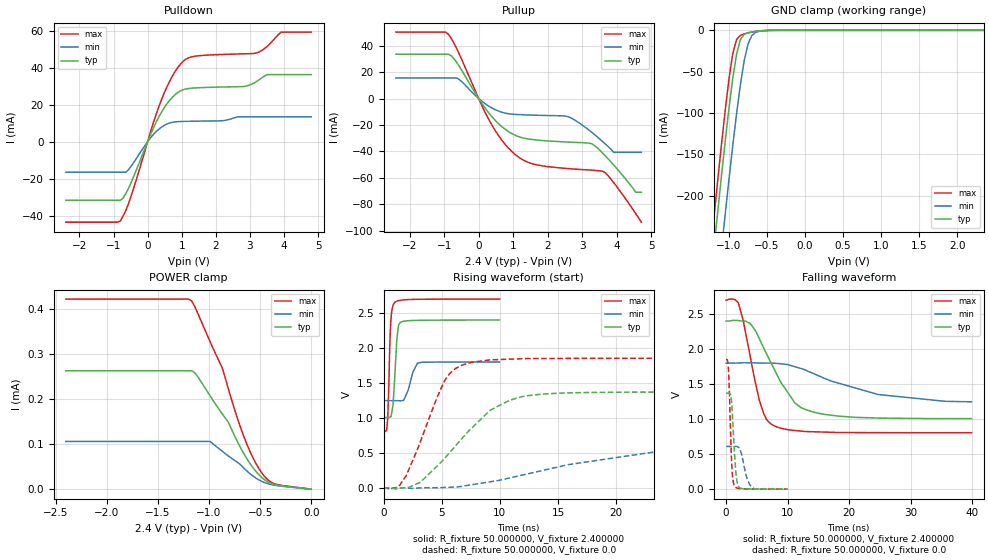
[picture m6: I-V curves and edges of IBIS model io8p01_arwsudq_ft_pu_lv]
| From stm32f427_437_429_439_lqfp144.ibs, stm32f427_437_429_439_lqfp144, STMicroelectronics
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|   Model io8p01_arwsudq_ft_pu_lv
[Model]  io8p01_arwsudq_ft_pu_lv
Model_type I/O
Polarity   Non-Inverting
Enable   Active-Low
Vinl =   0.720000V
Vinh =   1.680000V
Vmeas =  1.200000V
Cref =   50.000000pF
Rref =   100.000000M
Vref =   0.0V
C_comp   2.818400pF   2.774300pF   2.917100pF
[Temperature Range]   25.000000   0.125000k   -40.000000
[Pullup Reference]   2.400000V   1.800000V   2.700000V
[Pulldown Reference]   0.0V   0.0V   0.0V
[POWER Clamp Reference]   2.400000V   1.800000V   2.700000V
[GND Clamp Reference]   0.0V   0.0V   0.0V
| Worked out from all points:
|   slope of the pulldown table from 0 to 0.36 V, typ, clamps not added: 25 ohm
|   slope of the pullup table from 0 to 0.36 V, typ, clamps not added: 27.7 ohm
|   GND clamp passes 1 mA (typ) near -0.62 V on its own axis
|   rising waveform, R_fixture 50.000000, V_fixture 2.400000: 20-80 % time 290ps typ, 615ps min, 205ps max; typ from 1.01 V to 2.4 V
|   rising waveform, R_fixture 50.000000, V_fixture 0.0: 20-80 % time 4.71ns typ, 11.9ns min, 2.66ns max; typ from 0.001 V to 1.37 V
|   falling waveform, R_fixture 50.000000, V_fixture 2.400000: 20-80 % time 5.22ns typ, 11.3ns min, 2.74ns max; typ from 2.4 V to 1.01 V
|   falling waveform, R_fixture 50.000000, V_fixture 0.0: 20-80 % time 543ps typ, 1ns min, 410ps max; typ from 1.37 V to 0.001 V
[Pulldown]
|Voltage   I(typ)   I(min)   I(max)
-2.4V     -31.67mA   -16.51mA   -43.52mA
-800mV    -31.67mA   -16.51mA   -42.87mA
-480mV    -21.98mA   -13.17mA   -29.21mA
80mV      3.63mA     1.966mA    5.012mA
480mV     18.16mA    8.738mA    26.02mA
800mV     25.38mA    10.72mA    37.77mA
1.12V     28.53mA    11.02mA    44.6mA
2.8V      29.84mA    13.46mA    47.53mA
3.2V      32.6mA     13.46mA    48.03mA
3.52V     36.31mA    13.46mA    51.75mA
3.92V     36.31mA    13.46mA    59.29mA
4.8V      36.31mA    13.46mA    59.29mA
[Pullup]
|Voltage   I(typ)   I(min)   I(max)
-2.4V     33.5mA     15.56mA    50.23mA
-960mV    33.5mA     15.56mA    50.23mA
-560mV    24.27mA    14.3mA     33.51mA
320mV     -11.75mA   -6.207mA   -17.08mA
960mV     -26.47mA   -11.82mA   -40.02mA
1.52V     -30.88mA   -12.51mA   -49.05mA
2.56V     -32.88mA   -13.48mA   -52.9mA
3.28V     -34.19mA   -25.52mA   -54.17mA
3.6V      -41.32mA   -32.62mA   -54.98mA
3.92V     -50.33mA   -40.7mA    -63.65mA
4.56V     -70.9mA    -40.7mA    -87.11mA
4.72V     -70.9mA    -40.7mA    -93.5mA
[GND_clamp]
|Voltage   I(typ)   I(min)   I(max)
-2.4V     -1.425A    -1.509A    -1.395A
-1.25V    -311.8mA   -402mA     -274.5mA
-1.2V     -266mA     -356.2mA   -228.4mA
-1.15V    -220.9mA   -310.9mA   -183.1mA
-1.1V     -176.9mA   -266.3mA   -139mA
-1.05V    -134.3mA   -222.6mA   -97.01mA
-950mV    -57.81mA   -139.1mA   -27.86mA
-900mV    -28.73mA   -100.5mA   -11.04mA
-850mV    -11.29mA   -65.69mA   -6.054mA
-750mV    -2.852mA   -16.6mA    -3.179mA
-600mV    -750uA     -1.167mA   -738.5uA
2.35V     0A         0A         0A
[POWER_clamp]
|Voltage   I(typ)   I(min)   I(max)
-2.4V     263.2uA    106uA      422.4uA
-1.17V    263.2uA    106uA      418.5uA
-1.11V    250.1uA    106uA      391.1uA
-990mV    207.7uA    106uA      328.2uA
-870mV    167.2uA    84.17uA    269.6uA
-810mV    148.5uA    73.71uA    222.7uA
-660mV    79.21uA    47.09uA    117.6uA
-570mV    47.82uA    29.3uA     69.9uA
-510mV    31.66uA    20.4uA     45.18uA
-420mV    15.55uA    11.87uA    19.89uA
-360mV    10.34uA    8.845uA    12.09uA
0V        0A         0A         0A
[Ramp]
| variable   typ   min   max
dV/dt_r  0.82207/4.70989n   0.36536/11.91797n   1.11094/2.65517n
dV/dt_f  0.83604/5.22012n   0.32160/11.57067n   1.13651/2.74028n
R_load = 50.000000
[Rising Waveform]
R_fixture= 50.000000
V_fixture= 2.400000
V_fixture_min= 1.800000
V_fixture_max= 2.700000
|time   V(typ)   V(min)   V(max)
0s        1.007V     1.247V     805.8mV
340.3ps   1.007V     1.247V     975.4mV
600.6ps   1.017V     1.247V     2.337V
800.8ps   1.18V      1.247V     2.605V
961ps     1.604V     1.247V     2.653V
1.121ns   2.093V     1.247V     2.669V
1.261ns   2.305V     1.247V     2.676V
1.502ns   2.371V     1.247V     2.683V
2.923ns   2.395V     1.783V     2.696V
9.97ns    2.4V       1.8V       2.7V
[Rising Waveform]
R_fixture= 50.000000
V_fixture= 0.0
V_fixture_min= 0.0
V_fixture_max= 0.0
|time   V(typ)   V(min)   V(max)
0s        1.06mV     913.5uV    1.424mV
1.281ns   -8.248mV   1.007mV    20.35mV
1.922ns   3.767mV    -1.541mV   168.6mV
3.123ns   77.93mV    -442.3uV   645.2mV
5.205ns   415.5mV    5.78mV     1.518V
6.887ns   734.4mV    26.97mV    1.763V
9.209ns   1.114V     88.46mV    1.831V
12.57ns   1.322V     207.4mV    1.849V
24.5ns    1.37V      542.7mV    1.853V
39.88ns   1.371V     610.2mV    1.852V
[Falling Waveform]
R_fixture= 50.000000
V_fixture= 2.400000
V_fixture_min= 1.800000
V_fixture_max= 2.700000
|time   V(typ)   V(min)   V(max)
0s        2.4V       1.8V       2.7V
2.002ns   2.407V     1.801V     2.659V
4.004ns   2.358V     1.805V     1.86V
5.445ns   2.141V     1.801V     1.26V
6.486ns   1.949V     1.8V       1.011V
7.688ns   1.737V     1.799V     911.4mV
11.21ns   1.229V     1.748V     838mV
14.17ns   1.102V     1.652V     820.1mV
24.74ns   1.016V     1.351V     807.1mV
39.88ns   1.007V     1.247V     805.8mV
[Falling Waveform]
R_fixture= 50.000000
V_fixture= 0.0
V_fixture_min= 0.0
V_fixture_max= 0.0
|time   V(typ)   V(min)   V(max)
0s        1.371V     610.2mV    1.852V
380.4ps   1.371V     610.2mV    1.729V
880.9ps   1.264V     610mV      439.8mV
1.081ns   989.9mV    609.7mV    158mV
1.361ns   529mV      609.9mV    50.67mV
1.722ns   140.4mV    612mV      19.11mV
2.202ns   23.36mV    586.1mV    9.845mV
3.303ns   5.69mV     177.7mV    4.88mV
4.505ns   3.702mV    10.25mV    2.484mV
9.97ns    1.06mV     913.5uV    1.424mV
